(* Logix 5000 AddOnInstructionDefinition export MAM_Yaskawa; software revision 17.00 *)

TYPE Yaskawa_EIP_Servo :   // Yaskawa SigmaLogic Axis Structure v2.4.0
STRUCT
   O : Yaskawa_OUT_to_Servo;
   I : Yaskawa_IN_from_Servo;
   AOI_SB : Yaskawa_AOI_Status_Bits;
END_STRUCT
END_TYPE

TYPE Yaskawa_OUT_to_Servo :   // Structure of data sent out to the Yaskawa SigmaLogic controller v2.4.0
STRUCT
   b00_ServoOn : BOOL;   // Servo On
   b01_Stop : BOOL;   // Stops All Current Motion in Progress
   b02_Home : BOOL;   // Start Homing Process
   b03_MoveStart1 : BOOL;   // Start Current Motion
   b06_SuperImpose : BOOL;
   b07_ServoAlarmReset : BOOL;   // Servo Alarm Reset
   b08_ControllerAlarmReset : BOOL;   // SigmaLogic Alarm Reset
   b09_MoveStart2 : BOOL;   // Start Second Motion (Blended Move)
   b10_MoveAbort : BOOL;   // Abort Current Move
   b11_MovePause : BOOL;   // Pause Current Move
   b12_SeqPause : BOOL;   // Indexing Sequence Pause
   b13_SeqResume : BOOL;   // Indexing Sequence Resume
   b14_SeqCancel : BOOL;   // Indexing Sequence Cancel
   b15_AbsEncoderReset : BOOL;   // Absolute Encoder Reset
   b16_SeqStart : BOOL;   // Start Indexing Sequence
   b17_SeqEditSpeed : BOOL;   // Enter Edit Speed
   b18_SeqEditDistance : BOOL;   // Enter Distance Edit
   b19_PLSEnable : BOOL;   // Enable PLS execution
   b20_PLSActivateOutput1 : BOOL;   // Activate PLS output1 switch logic
   b21_PLSActivateOutput2 : BOOL;   // Activate PLS output2 switch logic
   b22_PLSActivateOutput3 : BOOL;   // Activate PLS output3 switch logic
   b23_PLSActivateOutput4 : BOOL;   // Activate PLS output4 switch logic
   b24_SetClock : BOOL;   // Set the remote controller clock with data provided by the PLC
   RebootController : BOOL;
   UseExternalEncoder : BOOL;   // Use External Encoder when executing MAHSP_Yaskawa
   b32_HeatbeatAnswer : BOOL;   // Heartbeat Answer
   BrakeBypassRequest : BOOL;
   SetFwdTorqueLimit : BOOL;
   SetRevTorqueLimit : BOOL;
   TorqueLimit : DINT;
   TorqueRamp : DINT;
   HomeMethod : INT;
   HomeSpeed : DINT;
   HomeAccDec : DINT;   // Home Move Acceleration/Deceleration Rate
   HomeBackOffDistance : DINT;
   HomeCreepSpeed : DINT;
   HomeCreepDistanceLimit : DINT;
   HomeCreepTimeLimit : DINT;
   HomeOffsetDistance : DINT;
   HomeOffsetSpeed : DINT;
   HomePostion : DINT;
   HomeTorque : DINT;
   HomeInputNo : DINT;
   HomeApproachTimeLimit : DINT;
   HomeApproachDistLimit : DINT;
   HomeDirection : INT;
   HomeSwitchMode : INT;
   MoveType : INT;
   MoveDirection : INT;
   MoveAccel1 : DINT;
   MoveAccel2 : DINT;
   MoveDecel1 : DINT;
   MoveDecel2 : DINT;
   MoveSpeed1 : DINT;
   MoveSpeed2 : DINT;
   MoveDistance1 : DINT;
   MoveDistance2 : DINT;
   MovePosition1 : DINT;
   MovePosition2 : DINT;
   RegistrationDistance : DINT;
   GearNumerator : DINT;
   GearDenominator : DINT;
   SuperImposeDistance : DINT;
   Resolution : INT;
   RegistrationDirection : INT;
   TuningLevel : INT;
   SequenceStep : INT;   // Staring Sequence Step Number
   SequenceEditStep : INT;   // Sequence Step Number to Edit
   FlagCommandBits1 : DINT;   // Flag Commands. 1..64 are General Flags, Bits 0..31 correspond to Flag 1..32
   FlagCommandBits2 : DINT;   // Flag Commands cont. 1..64 are General Flags, Bits 0..31 correspond to Flag 33..64
   DigitalOutCommandBits : DINT;   // Digital Output commands. Bits 0-7 correspond to CN13 Digital Outputs 0-7, used as Flag 73-80. Bits 8-10 correspond to CN1 Digital Outputs 0-2 used as Flag 88-90"
   SequenceEditSpeed : DINT;
   SequenceEditDistance : DINT;
   FeedRateOverride : INT;
   HSI_Enable : BOOL;
   HSI_MoveMode : BOOL;   // 0=Relative; 1=Moves per Cycle
   HSI_CalcMethod : BOOL;   // 0=Accel/Decel; 1=Time
   HSI_MoveDirection : BOOL;   // 0 = Negative; 1 = Positive
   HSI_TriggerFlag : INT;
   HSI_MovingFlag : INT;
   HSI_DwellingFlag : INT;
   HSI_DoneFlag : INT;
   HSI_MoveType : INT;   // 0=Single; 1=Repeat; 2=Repeat "x" times
   HSI_RepeatNumber : INT;
   HSI_Distance : DINT;
   HSI_Speed : DINT;
   HSI_Accel : DINT;
   HSI_MoveTime : DINT;
   HSI_DwellTime : DINT;
   PLS_OutputFlag1 : INT;
   PLS_OutputFlag2 : INT;
   PLS_OutputFlag3 : INT;
   PLS_OutputFlag4 : INT;
   PLS_OnPosition1 : DINT;
   PLS_OffPosition1 : DINT;
   PLS_OnPosition2 : DINT;
   PLS_OffPosition2 : DINT;
   PLS_OnPosition3 : DINT;
   PLS_OffPosition3 : DINT;
   PLS_OnPosition4 : DINT;
   PLS_OffPosition4 : DINT;
   PLS_OnCompensation1 : INT;
   PLS_OffCompensation1 : INT;
   PLS_OnCompensation2 : INT;
   PLS_OffCompensation2 : INT;
   PLS_OnCompensation3 : INT;
   PLS_OffCompensation3 : INT;
   PLS_OnCompensation4 : INT;
   PLS_OffCompensation4 : INT;
   RTC_Year : INT;
   RTC_Month : INT;
   RTC_Day : INT;
   RTC_Hour : INT;
   RTC_Min : INT;
   RTC_Sec : INT;
   StopDecel : DINT;
   AnalogOutput : INT;   // CN13, AO_01 [mV]
END_STRUCT
END_TYPE

TYPE Yaskawa_AOI_Status_Bits :   // Internal bits used to interlock Yaskawa AOI execution. v2.4.0
STRUCT
   MAM : BOOL;   // Move AOI Active
   MAJ : BOOL;   // Jog AOI Active
   MAB : BOOL;   // Blending AOI Active
   MAG : BOOL;   // Gearing AOI Active
   MAHSP : BOOL;   // Home SetPoint AOI Active
   MAH : BOOL;   // Homing AOI Active
   MSQE : BOOL;   // Sequence Edit AOI Active
   MSQR : BOOL;   // Sequence Run AOI Active
   MHSI : BOOL;   // High Speed Index AOI Active
   MSO : BOOL;   // Servo On
   MSF : BOOL;   // Servo Off
   MAFR : BOOL;   // Fault Reset
   MAS : BOOL;   // Servo Abort
   MTRQ : BOOL;   // Torque Mode Active
   MPLS : BOOL;   // PLS Active
   MCLK : BOOL;   // SetClock Active
   MSTL : BOOL;   // Set Torque Limit Active
   AOI_Permissive : BOOL;   // Permissive to Execute an AOI
END_STRUCT
END_TYPE

TYPE Yaskawa_IN_from_Servo :   // Structure of data coming from the Yaskawa SigmaLogic controller. v2.4.0
STRUCT
   AlarmText : STRING;   // ServoPack Alarm Code plus Text Description
   b00_Heartbeat : BOOL;
   b01_Alarm : BOOL;   // ServoPack Alarm
   b02_Warning : BOOL;   // ServoPack Warning
   b03_Ready : BOOL;   // ServoPack Ready
   b04_Enabled : BOOL;   // ServoPack Enabled ("Servo On")
   b05_StopComplete : BOOL;
   b06_HomeComplete : BOOL;
   b07_HomeBusy : BOOL;
   b08_HomeActive : BOOL;
   b09_HomeAborted : BOOL;
   b10_HomeError : BOOL;
   b11_MoveAbsComplete : BOOL;
   b12_MoveAbsBusy : BOOL;
   b13_MoveAbsActive : BOOL;
   b14_MoveAbsAborted : BOOL;
   b15_MoveAbsError : BOOL;
   b16_MoveRelComplete : BOOL;
   b17_MoveRelBusy : BOOL;
   b18_MoveRelActive : BOOL;
   b19_MoveRelAborted : BOOL;
   b20_MoveRelError : BOOL;
   b21_JogAtSpeed : BOOL;
   b22_JogBusy : BOOL;
   b23_JogActive : BOOL;
   b24_JogAborted : BOOL;
   b25_JogError : BOOL;
   b26_GearInSync : BOOL;
   b27_GearBusy : BOOL;
   b28_GearActive : BOOL;
   b29_GearAborted : BOOL;
   b30_GearError : BOOL;
   b32_MoveSuperComplete : BOOL;
   b33_MoveSuperBusy : BOOL;
   b34_MoveSuperActive : BOOL;
   b35_MoveSuperAborted : BOOL;
   b36_MoveSuperError : BOOL;
   b37_PowerCycleRequired : BOOL;
   b38_MoveBlend1Complete : BOOL;
   b39_MoveBlend1Busy : BOOL;
   b40_MoveBlend1Active : BOOL;
   b41_MoveBlend1Abort : BOOL;
   b42_MoveBlend1Error : BOOL;
   b43_MoveBlend2Complete : BOOL;
   b44_MoveBlend2Busy : BOOL;
   b45_MoveBlend2Active : BOOL;
   b46_MoveBlend2Abort : BOOL;
   b47_MoveBlend2Error : BOOL;
   b48_RegComplete : BOOL;
   b49_RegBusy : BOOL;
   b50_RegActive : BOOL;
   b51_RegAborted : BOOL;
   b52_RegError : BOOL;
   b53_ResetAbsEncoderActive : BOOL;
   b54_ResetAbsEncoderBusy : BOOL;
   b55_ResetAbsEncoderDone : BOOL;
   b56_ResetAbsEncoderError : BOOL;
   b57_SeqRunning : BOOL;
   b58_RegSensorNotReached : BOOL;
   b59_SeqEditError : BOOL;
   b60_SeqEditDone : BOOL;
   b61_TorqueAtTorque : BOOL;
   b62_TorqueBusy : BOOL;
   b63_TorqueActive : BOOL;
   b64_TorqueAborted : BOOL;
   b65_TorqueError : BOOL;
   b66_ControllerAlarm : BOOL;
   b67_ApplicationError : BOOL;
   b68_AxisAtStandStill : BOOL;
   b69_TestModeActive : BOOL;
   b70_ServoParamsOK : BOOL;
   b71_SetFwdTorqueLimitDone : BOOL;
   b72_SetRevTorqueLimitDone : BOOL;
   Position : DINT;
   Speed : DINT;
   Torque : DINT;
   HomeErrorID : INT;
   MoveAbsErrorID : INT;
   MoveRelErrorID : INT;
   JogErrorID : INT;
   GearErrorID : INT;
   MoveSuperErrorID : INT;
   ServoAlarmID : INT;
   ServoWarningID : INT;
   ControllerAlarmID : DINT;
   AxisGenAlarmID : DINT;
   MoveBlend1ErrorID : INT;
   MoveBlend2ErrorID : INT;
   ResetAbsEncoderErrorID : INT;
   FunctionBlockErrorID : INT;
   TorqueErrorID : INT;
   RegErrorID : INT;
   SeqCurrentStep : INT;
   FlagStatusBit1 : DINT;   // Flag Status. 1..64 are General Flags, Bits 0..31 correspond to Flag 1..32
   FlagStatusBit2 : DINT;   // Flag Status cont. 1..64 are General Flags, Bits 0..31 correspond to Flag 33..64
   IOStatusBits : DINT;   // Digital IO Status. Bits 0-7, CN13 Inputs 0-7, Used as Flag 65-72. Bits 8-15, CN13 Outputs 0-7, Used as Flag 73-80. Bits 16-22, CN1 Inputs 0-6, Used as Flag 81-87. Bits 23-25, CN1 Outputs 0-4, Used as Flag 88-92.
   HSI_Moving : BOOL;
   HSI_Dwelling : BOOL;
   HSI_Done : BOOL;
   HSI_Busy : BOOL;
   HSI_Error : BOOL;
   HSI_ErrorCode : INT;
   PLS_Running : BOOL;
   PLS_SwitchStatus1 : BOOL;
   PLS_SwitchStatus2 : BOOL;
   PLS_SwitchStatus3 : BOOL;
   PLS_SwitchStatus4 : BOOL;
   PLS_Busy : BOOL;
   PLS_Error : BOOL;
   PLS_ErrorCode : INT;
   SetClock_Done : BOOL;
   SetClock_Busy : BOOL;
   SetClock_Error : BOOL;
   SetClock_ErrorID : INT;
   SoftwareVersion : DINT;
   FirmwareVersion : DINT;
   CommandedPos : DINT;
   CommandedPosNonCyc : DINT;
   CommandedSpeed : DINT;
   Clock_Year : INT;
   Clock_Month : INT;
   Clock_Day : INT;
   Clock_Hour : INT;
   Clock_Minute : INT;
   Clock_Second : INT;
   AnalogInput : REAL;   // CN13, AI_01 [v]
   BrakeBypassActive : BOOL;
   ForwardTorqueLimit : DINT;
   ReverseTorqueLimit : DINT;
END_STRUCT
END_TYPE

ADD_ON_INSTRUCTION MAM_Yaskawa   (* revision 2.4 0, vendor Yaskawa America, Inc., ExecuteEnableInFalse *)
// Motion Axis Move
// Revision note:
// 2.4.0: No functional change
// 2.3.1: Moved unlatch of AOI_ON_LOCAL to bottom of EnableInFalse routine so that outputs will be on for at least 1 scan if one-shot on EN is used.
// 2.3.0: No functional change
// 2.0.0: Improved output operation and error code reporting. Improved interlocking with embedded code.
// 1.2.0: No functional change.
// Initial Release 9/10/2014
// Help:
// This AOI moves a servo axis to a position based on the motion profile parameters. Use the Motion Axis Move instruction to move to a specified position (absolute) or a specified distance (Relative), with or without registration.
VAR_IN_OUT
   Axis : Yaskawa_EIP_Servo; {required}
END_VAR
VAR_INPUT
   Move_Type : DINT; {required}   // 0 = Linear Absolute 1 = Incremental (Relative) 2 = Rotary Absolute, Shortest Path 3 = Rotary Absolute, Positive 4 = Rotary Absolute, Negative
   Position : REAL; {required}   // If Absolute: Target Position If Incremental (Relative): Distance to Move
   Speed : REAL; {required}   // Commanded Speed [unit/s]
   Accel_Rate : REAL; {required}   // Acceleration rate [unit/s/s]
   Decel_Rate : REAL; {required}   // Deceleration rate [unit/s/s]
   RegistrationUse : INT; {required}   // 0 = Disabled (Do Not use Registration Latch) 1 = Enabled (Arm the Registration Latch)
   Reg_Distance : REAL; {required}   // Registration Distance (Relative) [unit]
   Reg_Speed : REAL; {required}   // Registration Move Speed [unit/s]
   Reg_Accel : REAL; {required}   // Registration Move Acceleration rate [unit/s/s]
   Reg_Decel : REAL; {required}   // Registration Move Deceleration rate [unit/s/s]
END_VAR
VAR_OUTPUT
   EN : BOOL; {visible}   // A false-to-true transition has caused the AOI to execute
   DN : BOOL; {visible}   // Motion has been initiated
   IP : BOOL; {visible}   // The axis is Moving to the end Position ("In Process")
   ER : BOOL; {visible}   // An error has occured
   PC : BOOL; {visible}   // The axis has reached the end Position ("Position Completed")
   RegDN : BOOL; {visible}   // Registration move has been initiated
   RegIP : BOOL; {visible}   // The Axis is moving to the Registration Position
   RegER : BOOL; {visible}   // An error has occurred with the Registration Move
   RegPC : BOOL; {visible}   // The Axis has reached the Registration Position
   FLT_PRM : BOOL; {visible}   // Invalid parameter
   FLT_RDY : BOOL; {visible}   // The Servo is Not Ready
   FLT_BSY : BOOL; {visible}   // There is another AOI Active for this Axis
   MoveErrorCode : INT; {visible}   // Move Error Code for Absolute Moves
   RegErrorCode : INT; {visible}   // Registration Move Error Code
END_VAR
VAR
   AOI_ON_LOCAL : BOOL;
   Move_ABS : BOOL;
   Move_ABS_wREG : BOOL;
   Move_REL : BOOL;
   Move_REL_wREG : BOOL;
   OneShotRising1 : BOOL;
   ONS1 : BOOL;
   ONS2 : BOOL;
   ScaleFactor : DINT;
   Finished : BOOL;   // Function is Finished
   Execute_OS : BOOL;
END_VAR

ROUTINE EnableInFalse   (* ladder *)
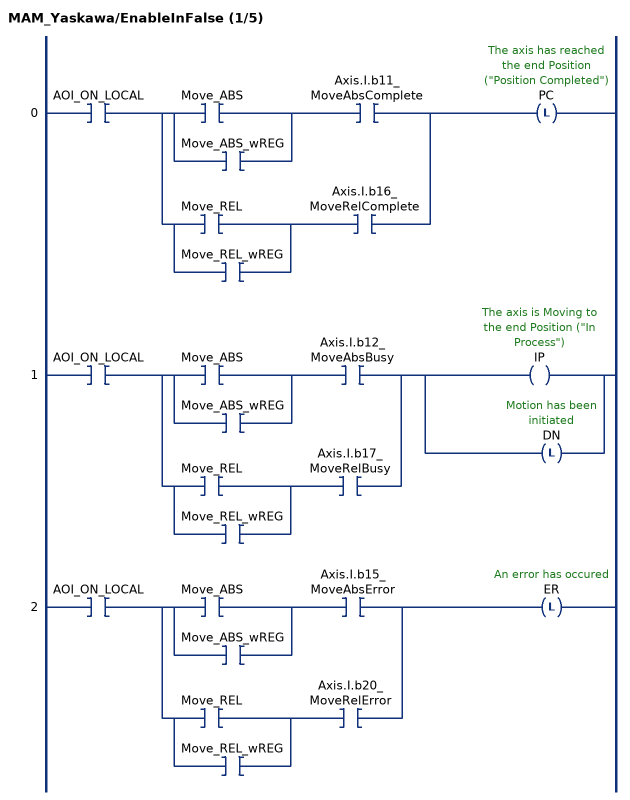
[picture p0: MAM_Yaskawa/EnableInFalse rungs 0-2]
   0: XIC(AOI_ON_LOCAL)[[XIC(Move_ABS) ,XIC(Move_ABS_wREG) ] XIC(Axis.I.b11_MoveAbsComplete) ,[XIC(Move_REL) ,XIC(Move_REL_wREG) ] XIC(Axis.I.b16_MoveRelComplete) ]OTL(PC);
   1: XIC(AOI_ON_LOCAL)[[XIC(Move_ABS) ,XIC(Move_ABS_wREG) ] XIC(Axis.I.b12_MoveAbsBusy) ,[XIC(Move_REL) ,XIC(Move_REL_wREG) ] XIC(Axis.I.b17_MoveRelBusy) ][OTE(IP) ,OTL(DN) ];
   2: XIC(AOI_ON_LOCAL)[[XIC(Move_ABS) ,XIC(Move_ABS_wREG) ] XIC(Axis.I.b15_MoveAbsError) ,[XIC(Move_REL) ,XIC(Move_REL_wREG) ] XIC(Axis.I.b20_MoveRelError) ]OTL(ER);
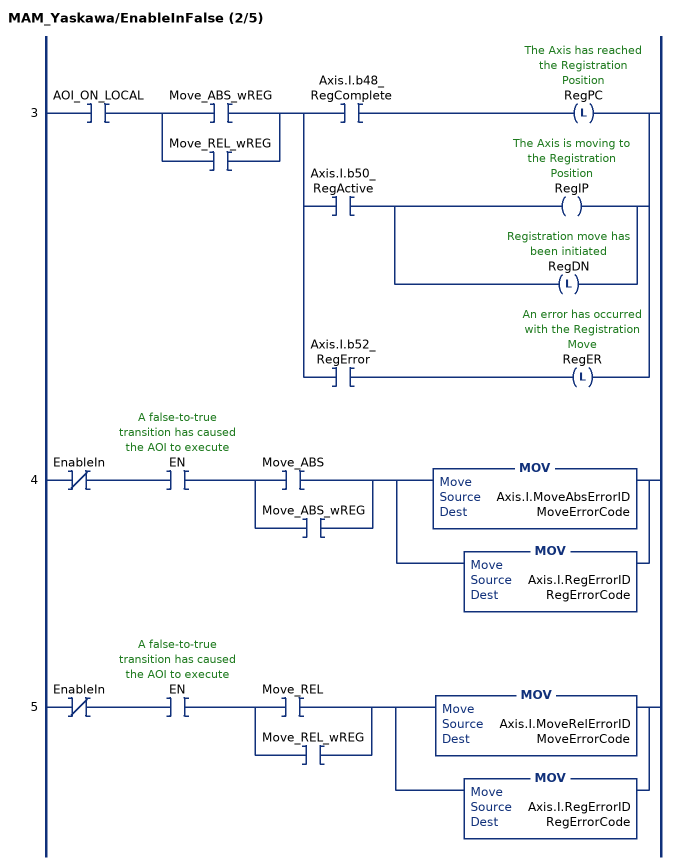
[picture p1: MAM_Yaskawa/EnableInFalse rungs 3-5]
   3: XIC(AOI_ON_LOCAL)[XIC(Move_ABS_wREG) ,XIC(Move_REL_wREG) ][XIC(Axis.I.b48_RegComplete) OTL(RegPC) ,XIC(Axis.I.b50_RegActive) [OTE(RegIP) ,OTL(RegDN) ] ,XIC(Axis.I.b52_RegError) OTL(RegER) ];
   4: XIO(EnableIn)XIC(EN)[XIC(Move_ABS) ,XIC(Move_ABS_wREG) ][MOV(Axis.I.MoveAbsErrorID,MoveErrorCode) ,MOV(Axis.I.RegErrorID,RegErrorCode) ];
   5: XIO(EnableIn)XIC(EN)[XIC(Move_REL) ,XIC(Move_REL_wREG) ][MOV(Axis.I.MoveRelErrorID,MoveErrorCode) ,MOV(Axis.I.RegErrorID,RegErrorCode) ];
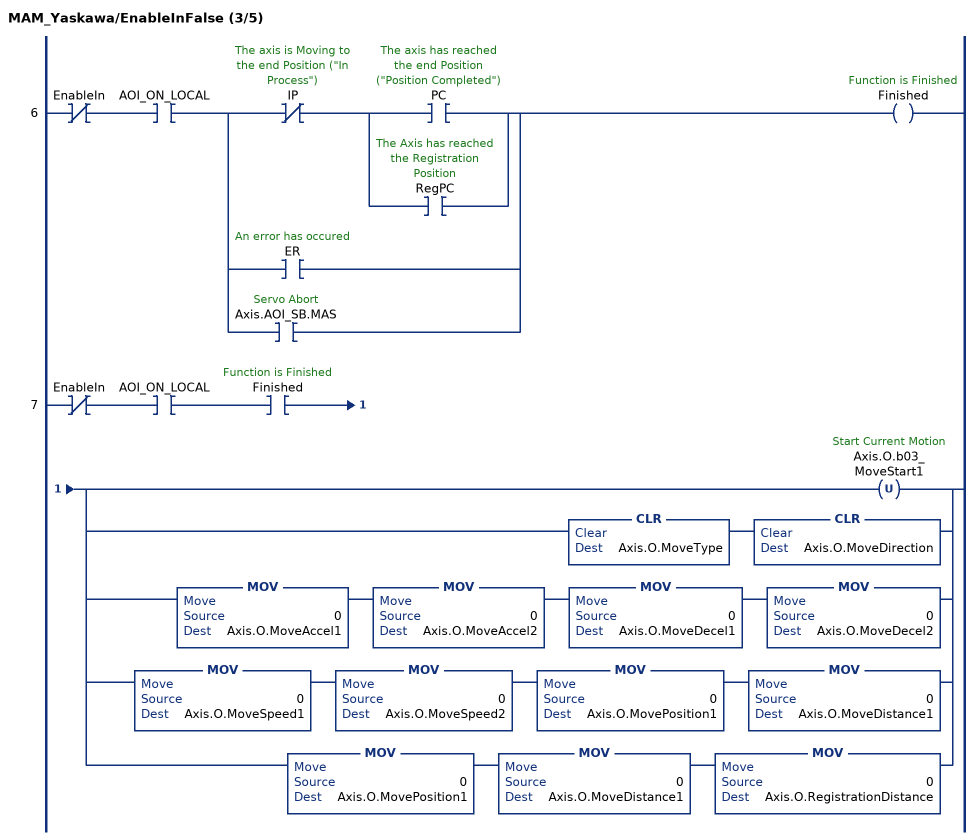
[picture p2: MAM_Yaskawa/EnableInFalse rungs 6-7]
   6: XIO(EnableIn)XIC(AOI_ON_LOCAL)[XIO(IP) [XIC(PC) ,XIC(RegPC) ] ,XIC(ER) ,XIC(Axis.AOI_SB.MAS) ]OTE(Finished);
   7: XIO(EnableIn)XIC(AOI_ON_LOCAL)XIC(Finished)[OTU(Axis.O.b03_MoveStart1) ,CLR(Axis.O.MoveType) CLR(Axis.O.MoveDirection) ,MOV(0,Axis.O.MoveAccel1) MOV(0,Axis.O.MoveAccel2) MOV(0,Axis.O.MoveDecel1) MOV(0,Axis.O.MoveDecel2) ,MOV(0,Axis.O.MoveSpeed1) MOV(0,Axis.O.MoveSpeed2) MOV(0,Axis.O.MovePosition1) MOV(0,Axis.O.MoveDistance1) ,MOV(0,Axis.O.MovePosition1) MOV(0,Axis.O.MoveDistance1) MOV(0,Axis.O.RegistrationDistance) ];
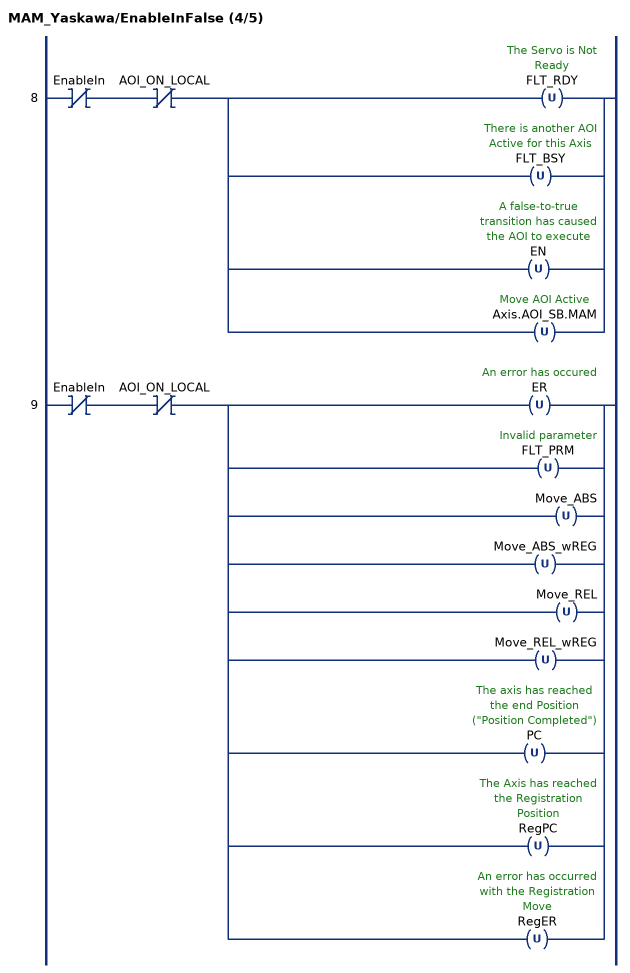
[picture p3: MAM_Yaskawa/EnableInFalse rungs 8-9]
   8: XIO(EnableIn)XIO(AOI_ON_LOCAL)[OTU(FLT_RDY) ,OTU(FLT_BSY) ,OTU(EN) ,OTU(Axis.AOI_SB.MAM) ];
   9: XIO(EnableIn)XIO(AOI_ON_LOCAL)[OTU(ER) ,OTU(FLT_PRM) ,OTU(Move_ABS) ,OTU(Move_ABS_wREG) ,OTU(Move_REL) ,OTU(Move_REL_wREG) ,OTU(PC) ,OTU(RegPC) ,OTU(RegER) ];
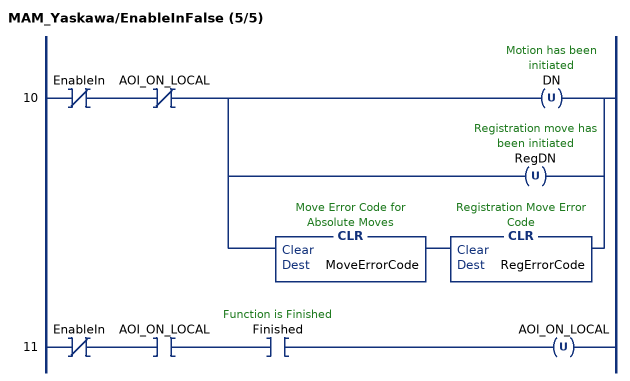
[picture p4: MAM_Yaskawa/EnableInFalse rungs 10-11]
   10: XIO(EnableIn)XIO(AOI_ON_LOCAL)[OTU(DN) ,OTU(RegDN) ,CLR(MoveErrorCode) CLR(RegErrorCode) ];
   11: XIO(EnableIn)XIC(AOI_ON_LOCAL)XIC(Finished)OTU(AOI_ON_LOCAL);
END_ROUTINE

ROUTINE Logic   (* ladder *)
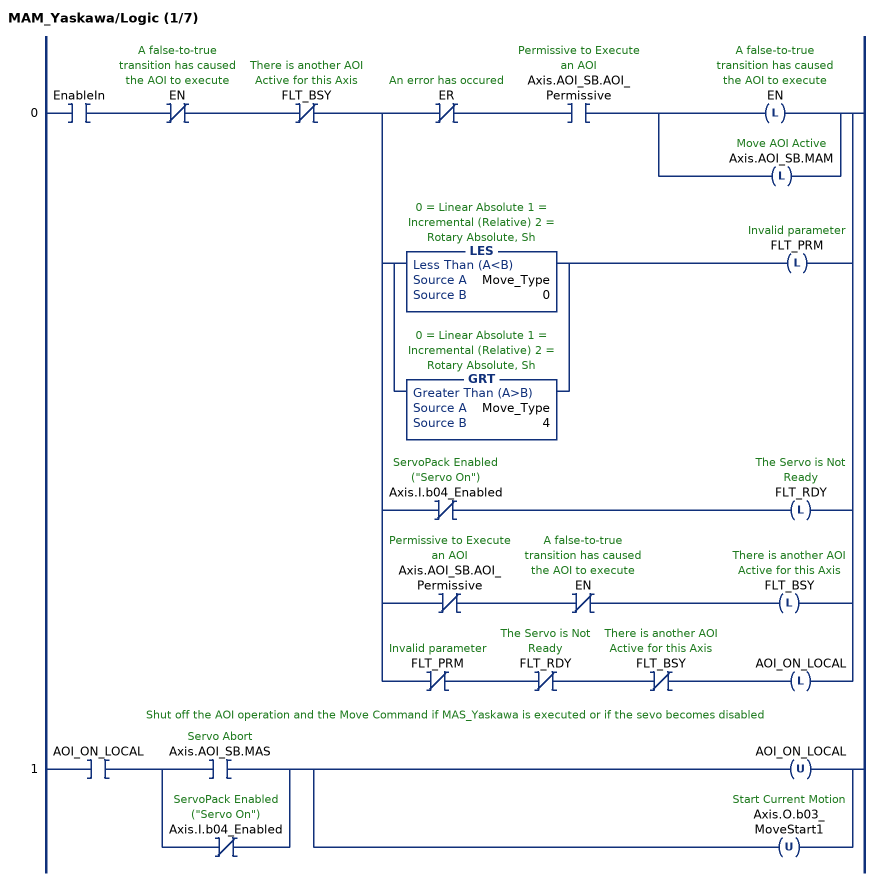
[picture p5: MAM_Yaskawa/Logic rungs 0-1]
   0: XIC(EnableIn)XIO(EN)XIO(FLT_BSY)[XIO(ER) XIC(Axis.AOI_SB.AOI_Permissive) [OTL(EN) ,OTL(Axis.AOI_SB.MAM) ] ,[LES(Move_Type,0) ,GRT(Move_Type,4) ] OTL(FLT_PRM) ,XIO(Axis.I.b04_Enabled) OTL(FLT_RDY) ,XIO(Axis.AOI_SB.AOI_Permissive) XIO(EN) OTL(FLT_BSY) ,XIO(FLT_PRM) XIO(FLT_RDY) XIO(FLT_BSY) OTL(AOI_ON_LOCAL) ];
   // Shut off the AOI operation and the Move Command if MAS_Yaskawa is executed or if the sevo becomes disabled
   1: XIC(AOI_ON_LOCAL)[XIC(Axis.AOI_SB.MAS) ,XIO(Axis.I.b04_Enabled) ][OTU(AOI_ON_LOCAL) ,OTU(Axis.O.b03_MoveStart1) ];
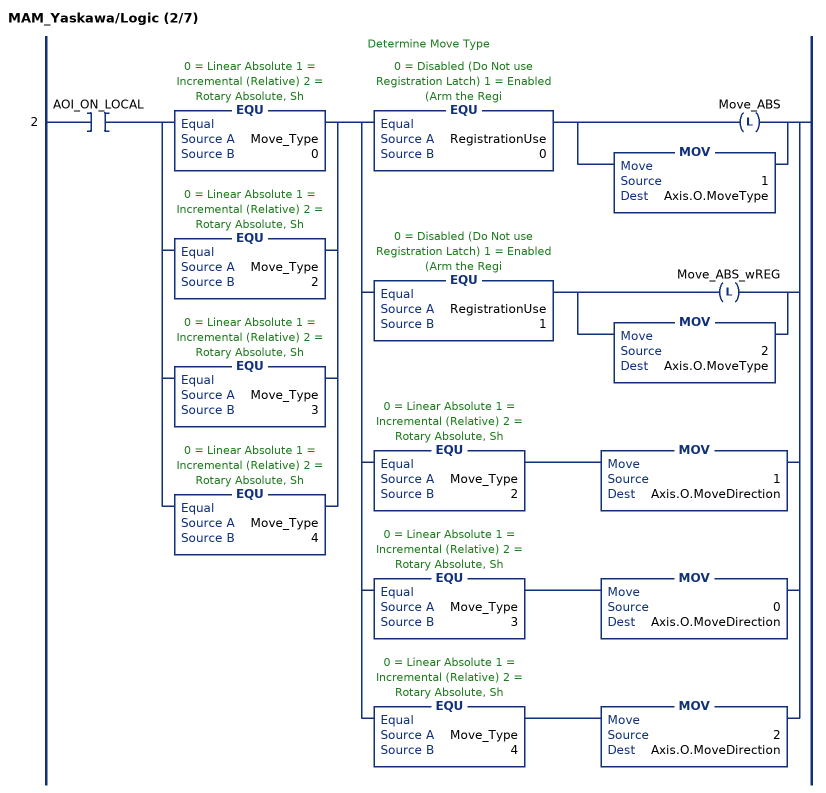
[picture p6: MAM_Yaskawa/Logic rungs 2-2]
   // Determine Move Type
   2: XIC(AOI_ON_LOCAL)[EQU(Move_Type,0) ,EQU(Move_Type,2) ,EQU(Move_Type,3) ,EQU(Move_Type,4) ][EQU(RegistrationUse,0) [OTL(Move_ABS) ,MOV(1,Axis.O.MoveType) ] ,EQU(RegistrationUse,1) [OTL(Move_ABS_wREG) ,MOV(2,Axis.O.MoveType) ] ,EQU(Move_Type,2) MOV(1,Axis.O.MoveDirection) ,EQU(Move_Type,3) MOV(0,Axis.O.MoveDirection) ,EQU(Move_Type,4) MOV(2,Axis.O.MoveDirection) ];
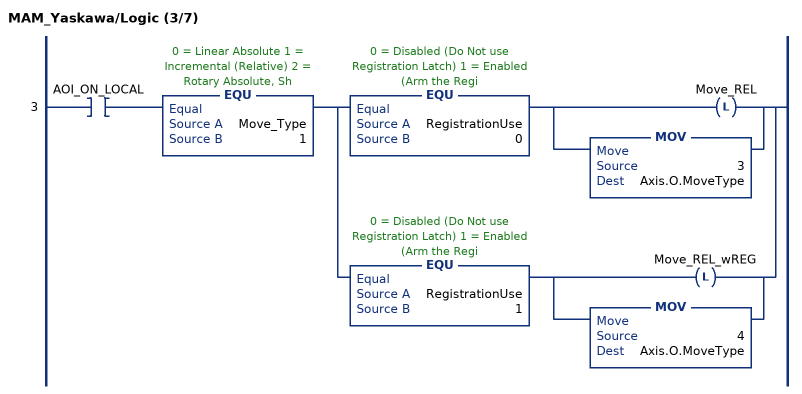
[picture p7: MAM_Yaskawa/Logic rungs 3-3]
   3: XIC(AOI_ON_LOCAL)EQU(Move_Type,1)[EQU(RegistrationUse,0) [OTL(Move_REL) ,MOV(3,Axis.O.MoveType) ] ,EQU(RegistrationUse,1) [OTL(Move_REL_wREG) ,MOV(4,Axis.O.MoveType) ] ];
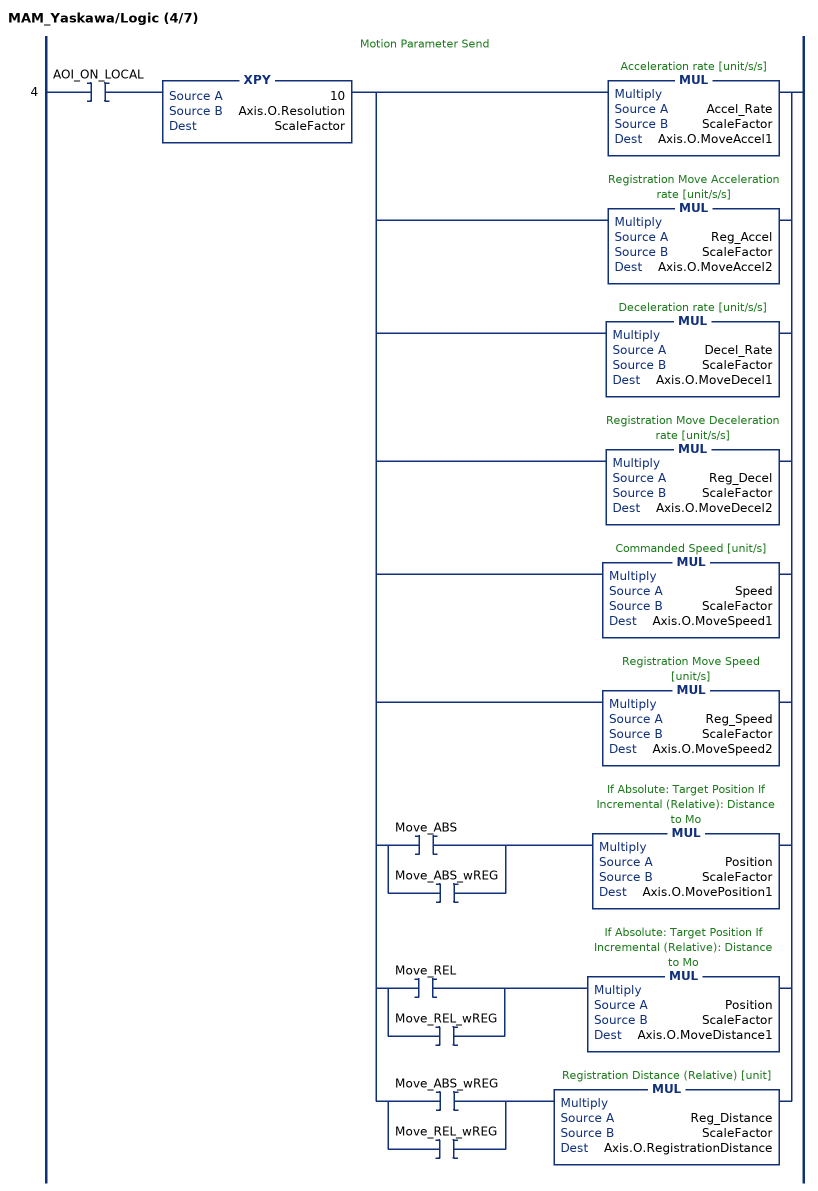
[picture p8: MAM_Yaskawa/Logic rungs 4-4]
   // Motion Parameter Send
   4: XIC(AOI_ON_LOCAL)XPY(10,Axis.O.Resolution,ScaleFactor)[MUL(Accel_Rate,ScaleFactor,Axis.O.MoveAccel1) ,MUL(Reg_Accel,ScaleFactor,Axis.O.MoveAccel2) ,MUL(Decel_Rate,ScaleFactor,Axis.O.MoveDecel1) ,MUL(Reg_Decel,ScaleFactor,Axis.O.MoveDecel2) ,MUL(Speed,ScaleFactor,Axis.O.MoveSpeed1) ,MUL(Reg_Speed,ScaleFactor,Axis.O.MoveSpeed2) ,[XIC(Move_ABS) ,XIC(Move_ABS_wREG) ] MUL(Position,ScaleFactor,Axis.O.MovePosition1) ,[XIC(Move_REL) ,XIC(Move_REL_wREG) ] MUL(Position,ScaleFactor,Axis.O.MoveDistance1) ,[XIC(Move_ABS_wREG) ,XIC(Move_REL_wREG) ] MUL(Reg_Distance,ScaleFactor,Axis.O.RegistrationDistance) ];
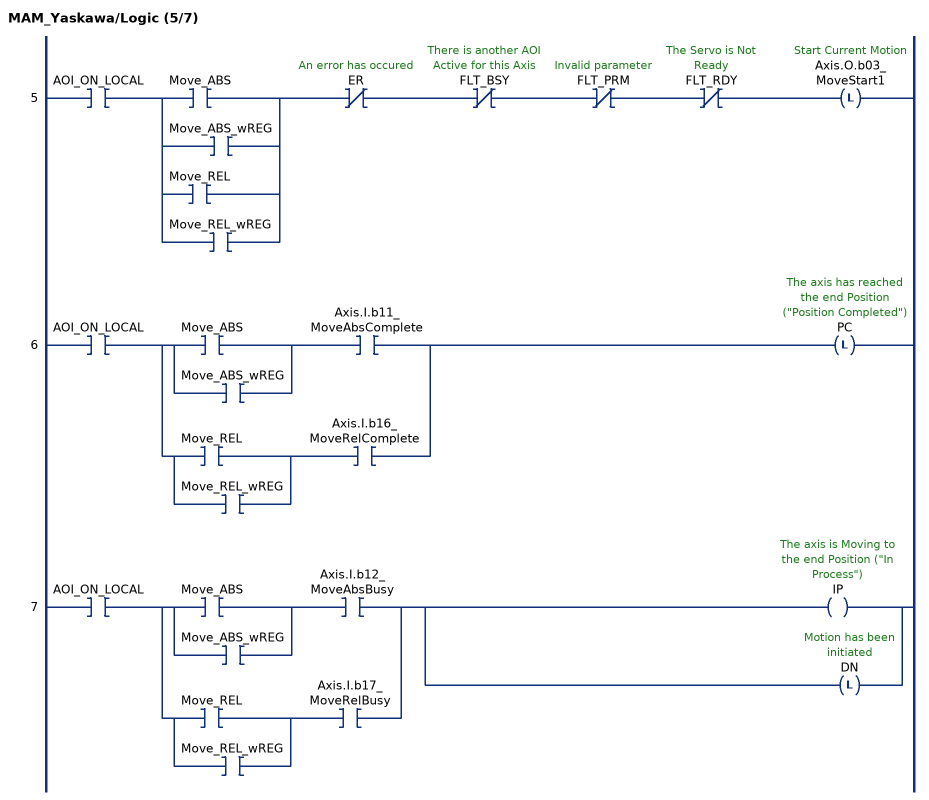
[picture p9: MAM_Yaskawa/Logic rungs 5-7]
   5: XIC(AOI_ON_LOCAL)[XIC(Move_ABS) ,XIC(Move_ABS_wREG) ,XIC(Move_REL) ,XIC(Move_REL_wREG) ]XIO(ER)XIO(FLT_BSY)XIO(FLT_PRM)XIO(FLT_RDY)OTL(Axis.O.b03_MoveStart1);
   6: XIC(AOI_ON_LOCAL)[[XIC(Move_ABS) ,XIC(Move_ABS_wREG) ] XIC(Axis.I.b11_MoveAbsComplete) ,[XIC(Move_REL) ,XIC(Move_REL_wREG) ] XIC(Axis.I.b16_MoveRelComplete) ]OTL(PC);
   7: XIC(AOI_ON_LOCAL)[[XIC(Move_ABS) ,XIC(Move_ABS_wREG) ] XIC(Axis.I.b12_MoveAbsBusy) ,[XIC(Move_REL) ,XIC(Move_REL_wREG) ] XIC(Axis.I.b17_MoveRelBusy) ][OTE(IP) ,OTL(DN) ];
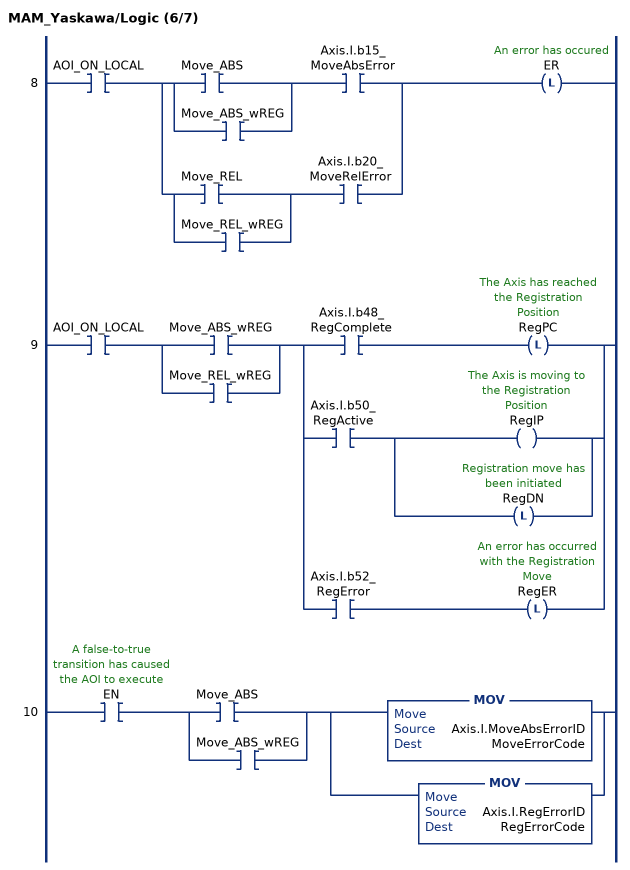
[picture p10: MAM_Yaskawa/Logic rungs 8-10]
   8: XIC(AOI_ON_LOCAL)[[XIC(Move_ABS) ,XIC(Move_ABS_wREG) ] XIC(Axis.I.b15_MoveAbsError) ,[XIC(Move_REL) ,XIC(Move_REL_wREG) ] XIC(Axis.I.b20_MoveRelError) ]OTL(ER);
   9: XIC(AOI_ON_LOCAL)[XIC(Move_ABS_wREG) ,XIC(Move_REL_wREG) ][XIC(Axis.I.b48_RegComplete) OTL(RegPC) ,XIC(Axis.I.b50_RegActive) [OTE(RegIP) ,OTL(RegDN) ] ,XIC(Axis.I.b52_RegError) OTL(RegER) ];
   10: XIC(EN)[XIC(Move_ABS) ,XIC(Move_ABS_wREG) ][MOV(Axis.I.MoveAbsErrorID,MoveErrorCode) ,MOV(Axis.I.RegErrorID,RegErrorCode) ];
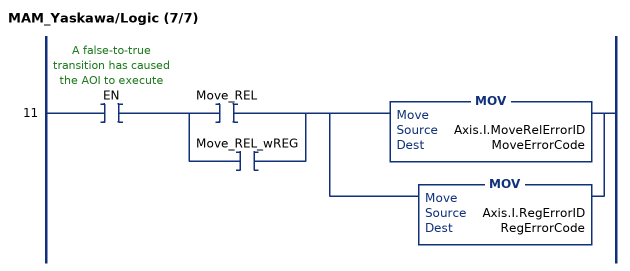
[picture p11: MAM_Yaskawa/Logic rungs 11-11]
   11: XIC(EN)[XIC(Move_REL) ,XIC(Move_REL_wREG) ][MOV(Axis.I.MoveRelErrorID,MoveErrorCode) ,MOV(Axis.I.RegErrorID,RegErrorCode) ];
END_ROUTINE
END_ADD_ON_INSTRUCTION
